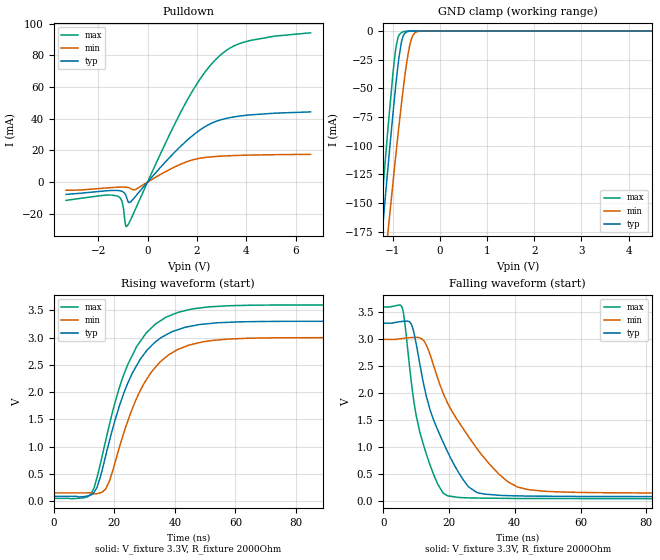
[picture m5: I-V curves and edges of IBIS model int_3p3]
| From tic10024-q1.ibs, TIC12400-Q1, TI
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|   int_3p3 Model
[Model]   int_3p3
Model_type   Open_drain
Polarity   Inverting
Vmeas = 1.65
Vref = 3.3
Cref = 2pF
Rref = 2000
|   typ   min   max
C_comp   3.99613E-12F   3.9413E-12F   4.05171E-12F
| Where nom  PVT is Nominal Process, 3.3V, 27C
|   Fast PVT is Strong Process,  3.6V, -40C
|   Slow PVT is Weak Process,   3.0V, 150C
[Voltage Range]   3.3   3   3.6
|Junction Temperature
[Temperature Range]   27   150   -40
[Pullup Reference]   3.3   3   3.6
[Pulldown Reference]   -0   -0   -0
[Power Clamp Reference]   3.3   3   3.6
[GND Clamp Reference]   0   0   0
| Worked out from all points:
|   slope of the pulldown table from 0 to 0.495 V, typ, clamps not added: 56.2 ohm
|   GND clamp passes 1 mA (typ) near -0.71 V on its own axis
|   falling waveform, V_fixture 3.3V, R_fixture 2000Ohm: 20-80 % time 10.3ns typ, 16.1ns min, 6.44ns max; typ from 3.3 V to 0.088 V
|   rising waveform, V_fixture 3.3V, R_fixture 2000Ohm: 20-80 % time 12.6ns typ, 12.9ns min, 12.3ns max; typ from 0.088 V to 3.3 V
[Pulldown]
|   Voltage   I(typ)   I(min)   I(max)
-3.3V     -7.779mA   -5.186mA   -11.56mA
-1.201V   -5.31mA    -3.225mA   -8.963mA
-1.033V   -5.86mA    -3.153mA   -12.23mA
-864.6mV  -8.902mA   -3.25mA    -28.12mA
-785.4mV  -12.44mA   -3.445mA   -26.84mA
-676.5mV  -12.37mA   -4.114mA   -23.58mA
-488.4mV  -9.026mA   -4.673mA   -17.02mA
1.422V    23.84mA    11.84mA    46.48mA
2.66V     37.67mA    16.06mA    75.8mA
3.204V    40.3mA     16.58mA    83.36mA
3.897V    42.05mA    16.96mA    88.4mA
6.6V      44.36mA    17.54mA    94.33mA
[GND Clamp]
|   Voltage   I(typ)   I(min)   I(max)
-3.3V     -1.163A    -1.109A    -1.199A
-1.33V    -227.8mA   -272.9mA   -200.9mA
-1.162V   -147.8mA   -201.7mA   -115.6mA
-1.092V   -115.8mA   -172.9mA   -81.74mA
-993.3mV  -71.85mA   -132.4mA   -36.88mA
-924mV    -43.54mA   -104.9mA   -12.68mA
-864.6mV  -22.65mA   -82.15mA   -3.477mA
-785.4mV  -5.284mA   -53.63mA   -798.7uA
-706.2mV  -878.6uA   -28.74mA   -65.81uA
-627mV    -102.5uA   -10.71mA   -2.274uA
-458.7mV  -280.5nA   -344.2uA   0A
6.6V      0A         0A         0A
[POWER Clamp]
|   Voltage   I(typ)   I(min)   I(max)
-3.3V     0A         0A         0A
0V        0A         0A         0A
6.6V      0A         0A         0A
[Ramp]
R_load = 2000
|   typ   min   max
dV/dt_r   1.92693/1.25901e-08   1.7095/1.28661e-08   2.12924/1.23419e-08
dV/dt_f   1.92693/1.03257e-08   1.7095/1.61228e-08   2.12924/6.44066e-09
[Falling Waveform]
V_fixture = 3.3V
V_fixture_min = 3V
V_fixture_max = 3.6V
R_fixture = 2000Ohm
C_fixture = 0F
|   Time   V(typ)   V(min)   V(max)
0s        3.3V       3V         3.6V
5.67ns    3.332V     3.016V     3.604V
8.454ns   3.292V     3.034V     2.257V
9.993ns   2.927V     3.038V     1.601V
13.3ns    1.908V     2.869V     842.7mV
19.63ns   912.8mV    1.814V     103.4mV
28.5ns    164mV      979.6mV    62.72mV
37.92ns   107.7mV    363.2mV    56.85mV
44.42ns   99.89mV    215.9mV    54.63mV
200ns     88.45mV    150.8mV    51.26mV
[Rising Waveform]
V_fixture = 3.3V
V_fixture_min = 3V
V_fixture_max = 3.6V
R_fixture = 2000Ohm
C_fixture = 0F
|   Time   V(typ)   V(min)   V(max)
0s        88.45mV    150.8mV    51.26mV
12.27ns   113.6mV    150.7mV    126.2mV
14.26ns   250mV      136.8mV    432.3mV
17.19ns   846.7mV    227.6mV    1.124V
21.44ns   1.707V     945.1mV    2.047V
27.36ns   2.488V     1.888V     2.837V
32.38ns   2.86V      2.381V     3.185V
41.07ns   3.148V     2.785V     3.465V
64.52ns   3.292V     2.989V     3.594V
200ns     3.3V       3V         3.6V
